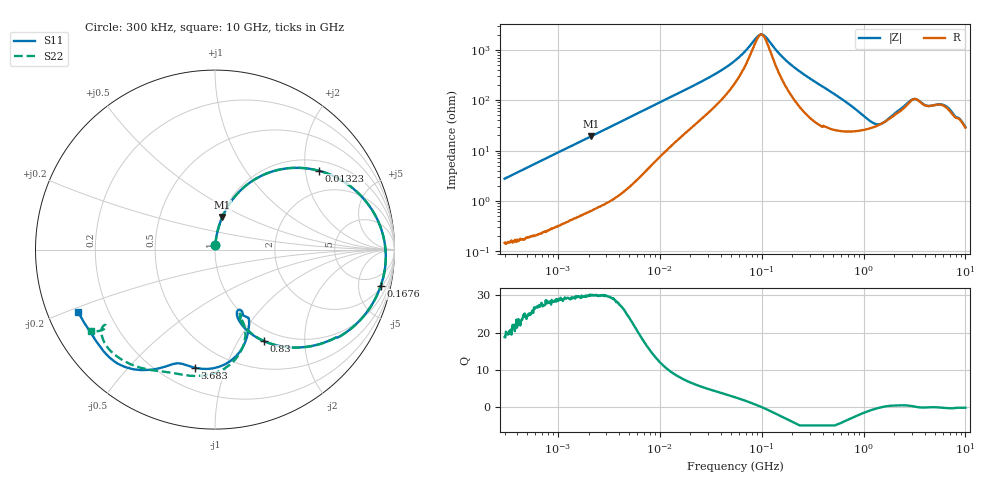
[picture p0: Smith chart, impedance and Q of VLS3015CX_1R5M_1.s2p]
! S-Parameter Data Generated by TDK Corporation
! Copyright(C) 2020 TDK Corporation.
! All Rights Reserved.
! TDK P/N: VLS3015CX-1R5M-1 (Inductor)
! Property: L=1.5uH at 1MHz
! Size(LxWxT): 3x3x1.5mm
! Model Type: s2p (Touchstone File Format Version 1.0)
! Frequency: DC=Yes Start=0.3MHz Stop=10000MHz 802points Log-sweep
! Model Generated on Aug. 18, 2020
! Port Assignments:
!  1 ---@@@--- 2
! Applicable Conditions:
!  Temperature = 25 degC
!  DC Bias Current = 0 A
!  Small Signal Operation
! Terms and conditions regarding TDK Simulation Models
! (1)This simulation model is being provided solely for informational purposes. Please refer to the specifications of the products in terms of detailed characteristics of such products.
! (2)In no event shall TDK Corporation of any of its subsidiaries be liable for any loss or damage arising, directly or indirectly,
!  From any information contained in this simulation model, including, but not limited to loss or damages arising from any inaccuracies, omissions or errors in connection with such information.
! (3)Any and all copyrights on this simulation model are owned by TDK Corporation.
!  Duplication or redistribution of this simulation model without prior written permission from TDK Corporation is prohibited.
! (4)This simulation model is subject to any modification or change without any prior notice.
! (5)Neither TDK Corporation nor any of its subsidiaries shall make any warranty, express or implied,
!  Including but not limited to the correctness, implied warranties of merchantability and fitness for a particular purpose with respect to this simulation models.
! (6)The use of this simulation model shall be deemed to have consented to the terms and conditions hereof.
# Hz S MA R 50
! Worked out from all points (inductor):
!   801 points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, 300 kHz to 10 GHz, reference 50 ohm
!   read as one part in series: L = 1.47 uH near 318.3 kHz
!   highest Q = 30 at 2.114 MHz (marker M1), where L = 1.44 uH
!   self-resonance near 98.84 MHz
!   S11 on the Smith chart (normalised r, x): 300 kHz: 1.00, +0.06; 13.23 MHz: 1.28, +2.38; 167.6 MHz: 2.29, -8.68; 830 MHz: 0.84, -1.30; 3.683 GHz: 0.33, -0.79; 10 GHz: 0.09, -0.22
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300000  0.02805 85.7  0.9981 -1.6  0.998 -1.6  0.02785 85.5
1713600  0.1523 79.3  0.9833 -8.8  0.9831 -8.8  0.1524 79.3
2114273  0.1861 77.3  0.9765 -10.8  0.9762 -10.8  0.1861 77.3
4673027  0.3822 65.1  0.9091 -22.6  0.9089 -22.6  0.3822 65.1
9671944  0.6328 46.0  0.7252 -39.4  0.7251 -39.4  0.6328 46.0
1.322782e7  0.7282 37.1  0.6112 -46.7  0.6111 -46.7  0.7282 37.0
3.031424e7  0.8852 17.3  0.3172 -60.9  0.3171 -60.9  0.8853 17.2
5.477226e7  0.934 6.8  0.1541 -62.1  0.1541 -62.1  0.934 6.8
9.914192e7  0.9525 -2.7  0.04746 -1.7  0.04743 -1.8  0.9526 -2.7
1.112655e8  0.9532 -4.6  0.05475 27.4  0.05473 27.4  0.9532 -4.7
1.6757e8  0.9454 -12.3  0.1435 59.3  0.1435 59.3  0.9454 -12.4
3.126428e8  0.8882 -28.0  0.3403 52.9  0.3402 52.9  0.8883 -28.1
5.225392e8  0.7587 -45.1  0.5261 34.5  0.526 34.5  0.7589 -45.2
8.299813e8  0.5799 -61.8  0.6616 11.9  0.6616 11.9  0.5815 -61.5
1.24442e9  0.4216 -71.2  0.7049 -11.6  0.7049 -11.6  0.43 -70.0
1.767019e9  0.3645 -67.2  0.6466 -35.2  0.6465 -35.3  0.388 -68.4
2.629198e9  0.5499 -72.7  0.4663 -59.8  0.4662 -59.8  0.492 -69.9
3.050901e9  0.6337 -83.5  0.3684 -62.9  0.3684 -63.0  0.6116 -78.4
3.682634e9  0.6668 -99.8  0.3372 -60.0  0.337 -60.0  0.706 -95.9
6.576072e9  0.8212 -126.9  0.2191 -81.5  0.2191 -81.4  0.7978 -128.0
8.211115e9  0.8376 -140.3  0.1935 -85.7  0.1937 -85.7  0.7533 -145.6
1e10  0.8373 -155.5  0.1895 -90.3  0.1895 -90.3  0.8279 -146.6
